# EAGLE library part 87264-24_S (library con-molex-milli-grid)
RECEPTACAL
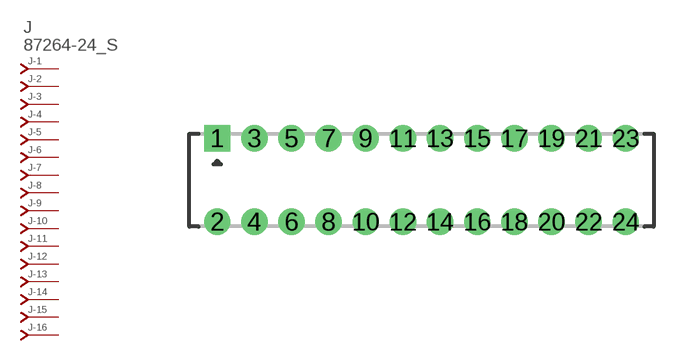
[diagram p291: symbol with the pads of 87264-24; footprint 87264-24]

Designator prefix J; gates -1=J-NV -2=J-N -3=J-N -4=J-N -5=J-N -6=J-N -7=J-N -8=J-N -9=J-N -10=J-N -11=J-N -12=J-N -13=J-N -14=J-N -15=J-N -16=J-N -17=J-N -18=J-N -19=J-N -20=J-N -21=J-N -22=J-N -23=J-N -24=J-N

## 87264-24_S  [87264-24]
1  -1:J  pas
2  -2:J  pas
3  -3:J  pas
4  -4:J  pas
5  -5:J  pas
6  -6:J  pas
7  -7:J  pas
8  -8:J  pas
9  -9:J  pas
10  -10:J  pas
11  -11:J  pas
12  -12:J  pas
13  -13:J  pas
14  -14:J  pas
15  -15:J  pas
16  -16:J  pas
17  -17:J  pas
18  -18:J  pas
19  -19:J  pas
20  -20:J  pas
21  -21:J  pas
22  -22:J  pas
23  -23:J  pas
24  -24:J  pas

## Footprint 87264-24 (pad centres in mm)
RECEPTACAL Dual Row, Side Entry
drill 0.914 square: 1 -11,2.25
drill 0.914: 2 -11,-2.25; 3 -9,2.25; 4 -9,-2.25; 5 -7,2.25; 6 -7,-2.25; 7 -5,2.25; 8 -5,-2.25; 9 -3,2.25; 10 -3,-2.25; 11 -1,2.25; 12 -1,-2.25; 13 1,2.25; 14 1,-2.25; 15 3,2.25; 16 3,-2.25; 17 5,2.25; 18 5,-2.25; 19 7,2.25; 20 7,-2.25; 21 9,2.25; 22 9,-2.25; 23 11,2.25; 24 11,-2.25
